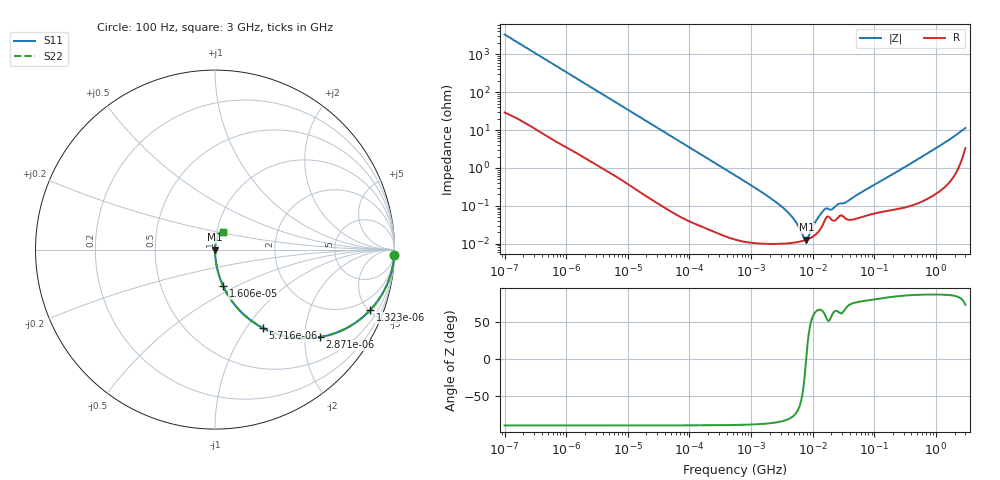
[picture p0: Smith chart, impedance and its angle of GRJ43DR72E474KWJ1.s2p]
!Murata Part Number: GRJ43DR72E474KWJ1
!These Parameters are Measured in Series Mode Connection
!Data Generated on Jun 19, 2026
!  o--ll--o
!Port1  Port2
!  o------o
!Operation Temp=25[degC], DC Bias Voltage=0[V]
!Freq. Start=100[Hz] Stop=3[GHz] 401[Steps]
# Hz S RI R 50
!Freq.(Hz) S11(Real) S11(Imag) S21(Real) S21(Imag) S12(Real) S12(Imag) S22(Real) S22(Imag)
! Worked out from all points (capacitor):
!   401 points, 100 Hz to 3 GHz, reference 50 ohm
!   read as one part in series: C = 477 nF near 109 Hz
!   lowest |Z| = 12.8 mohm at 7.898 MHz (marker M1)
!   series resonance near 7.822 MHz, so ESL is about 870 pH
!   S11 on the Smith chart (normalised r, x): 100 Hz: 2, -67; 1.323 kHz: 1.05, -5.13; 2.871 kHz: 1.03, -2.38; 5.716 kHz: 1.01, -1.20; 16.06 kHz: 1.00, -0.43; 3 GHz: 1.07, +0.22
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100  0.9988 -0.0299  0.00116 0.0299  0.00116 0.0299  0.9988 -0.0299
414  0.984 -0.1208  0.016 0.1208  0.016 0.1208  0.984 -0.1208
1323  0.8654 -0.3361  0.1346 0.3361  0.1346 0.3361  0.8654 -0.3361
1788  0.7808 -0.4084  0.2192 0.4084  0.2192 0.4084  0.7808 -0.4084
2871  0.5844 -0.4874  0.4156 0.4874  0.4156 0.4874  0.5844 -0.4874
5716  0.2668 -0.4368  0.7332 0.4368  0.7332 0.4368  0.2668 -0.4368
9178  0.1259 -0.3263  0.8741 0.3263  0.8741 0.3263  0.1259 -0.3263
16060  0.0461 -0.2046  0.9539 0.2046  0.9539 0.2046  0.0461 -0.2046
31977  0.0127 -0.107  0.9873 0.107  0.9873 0.107  0.0127 -0.107
547723  0.000169 -0.0064  0.9998 0.0064  0.9998 0.0064  0.000169 -0.0064
3339322  0.000101 -0.000867  0.9999 0.000867  0.9999 0.000867  0.000101 -0.000867
4919190  0.000107 -0.000437  0.9999 0.000437  0.9999 0.000437  0.000107 -0.000437
7246509  0.000121 -7.01e-05  0.9999 7.01e-05  0.9999 7.01e-05  0.000121 -7.01e-05
7897951  0.000127 9.1e-06  0.9999 -9.1e-06  0.9999 -9.1e-06  0.000127 9.1e-06
9794414  0.00015 0.000213  0.9999 -0.000213  0.9999 -0.000213  0.00015 0.000213
1.268047e7  0.000217 0.000487  0.9998 -0.000487  0.9998 -0.000487  0.000217 0.000487
1.572531e7  0.000415 0.000706  0.9996 -0.000706  0.9996 -0.000706  0.000415 0.000706
2.035898e7  0.000425 0.000685  0.9996 -0.000685  0.9996 -0.000685  0.000425 0.000685
2.635803e7  0.000513 0.001  0.9995 -0.001  0.9995 -0.001  0.000513 0.001
3.412477e7  0.000464 0.00113  0.9995 -0.00113  0.9995 -0.00113  0.000464 0.00113
1.751444e8  0.000786 0.00599  0.9992 -0.00599  0.9992 -0.00599  0.000786 0.00599
3e9  0.043 0.1003  0.957 -0.1003  0.957 -0.1003  0.043 0.1003
